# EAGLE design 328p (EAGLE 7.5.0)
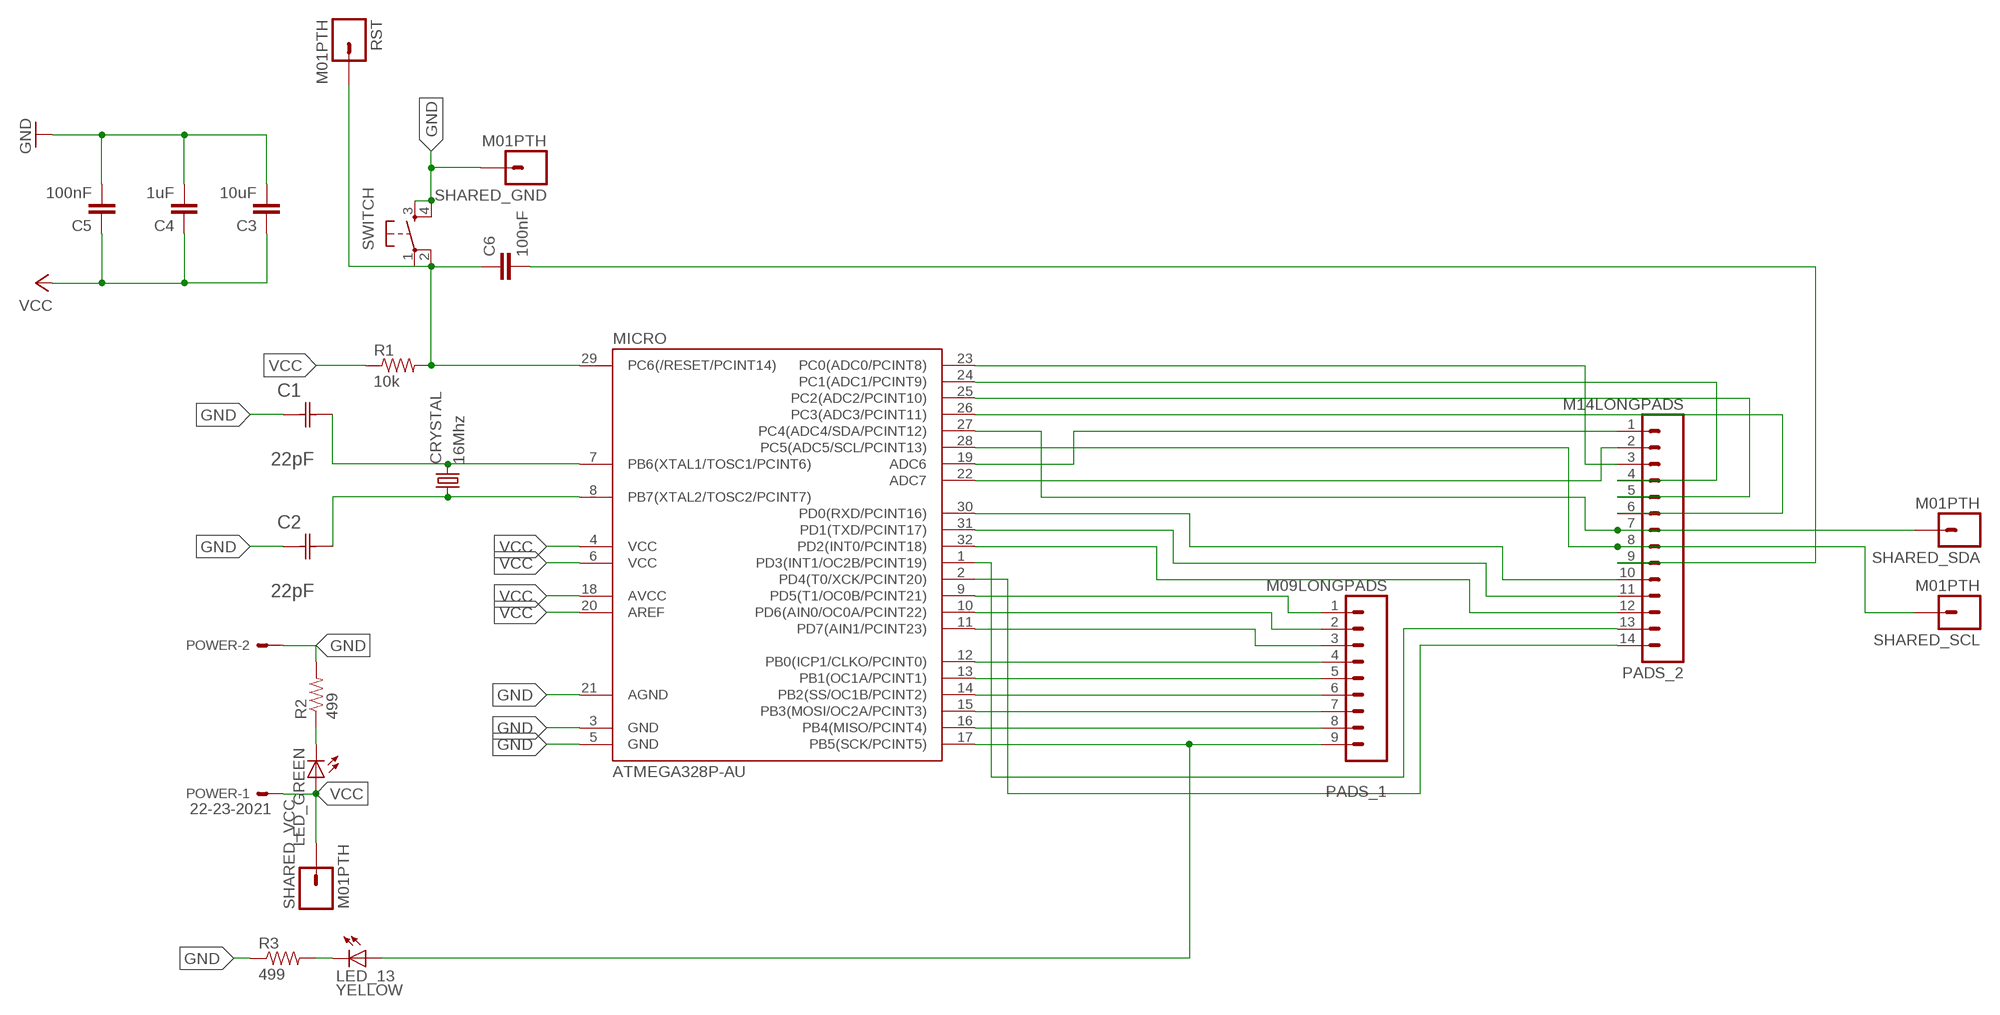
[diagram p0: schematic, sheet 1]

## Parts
C1  22pF  0612ZC225MAT2A  [CAPC3216X178N]
C2  22pF  0612ZC225MAT2A  [CAPC3216X178N]
C3  10uF  CAP1206  [1206]
C4  1uF  CAP1206  [1206]
C5  100nF  CAP1206  [1206]
C6  100nF  CAP1206  [1206]
CRYSTAL  16Mhz  CSM-7X-DU  [CSM-7X-DU]
LED_13  YELLOW  LED1206  [1206]
LED_GREEN  LED1206  [1206]
MICRO  ATMEGA328P-AU  ATMEGA48/88/168-AU  [TQFP32-08]
PADS_1  M09LONGPADS  [1X09_LONGPADS]
PADS_2  M14LONGPADS  [1X14-LONGPADS]
POWER  22-23-2021  [22-23-2021]
R1  10k  RESISTOR1206  [1206]
R2  499  RESISTOR1206  [1206]
R3  499  RESISTOR1206  [1206]
RST  M01PTH  [1X01]
SHARED_GND  M01PTH  [1X01]
SHARED_SCL  M01PTH  [1X01]
SHARED_SDA  M01PTH  [1X01]
SHARED_VCC  M01PTH  [1X01]
SWITCH  6MM_SWITCH6MM_SWITCH  [6MM_SWITCH]

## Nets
GND: C1.1(C1) C2.1(C1) C3.2 C4.2 C5.2 MICRO.3(GND) MICRO.5(GND) MICRO.21(AGND) POWER.2 R2.2 R3.1 SHARED_GND.1 SWITCH.3(S) SWITCH.4(S1)
N$1: MICRO.9(PD5(T1/OC0B/PCINT21)) PADS_1.1
N$2: C1.2(C2) CRYSTAL.2 MICRO.7(PB6(XTAL1/TOSC1/PCINT6))
N$3: C6.2 PADS_2.9
N$4: MICRO.10(PD6(AIN0/OC0A/PCINT22)) PADS_1.2
N$5: MICRO.11(PD7(AIN1/PCINT23)) PADS_1.3
N$6: MICRO.12(PB0(ICP1/CLKO/PCINT0)) PADS_1.4
N$7: MICRO.13(PB1(OC1A/PCINT1)) PADS_1.5
N$8: MICRO.14(PB2(SS/OC1B/PCINT2)) PADS_1.6
N$9: C2.2(C2) CRYSTAL.1 MICRO.8(PB7(XTAL2/TOSC2/PCINT7))
N$10: MICRO.15(PB3(MOSI/OC2A/PCINT3)) PADS_1.7
N$11: MICRO.16(PB4(MISO/PCINT4)) PADS_1.8
N$12: LED_13.1(A) MICRO.17(PB5(SCK/PCINT5)) PADS_1.9
N$13: MICRO.19(ADC6) PADS_2.1
N$14: MICRO.22(ADC7) PADS_2.2
N$15: MICRO.23(PC0(ADC0/PCINT8)) PADS_2.3
N$16: MICRO.24(PC1(ADC1/PCINT9)) PADS_2.4
N$17: MICRO.25(PC2(ADC2/PCINT10)) PADS_2.5
N$18: MICRO.26(PC3(ADC3/PCINT11)) PADS_2.6
N$19: MICRO.27(PC4(ADC4/SDA/PCINT12)) PADS_2.7 SHARED_SDA.1
N$20: MICRO.30(PD0(RXD/PCINT16)) PADS_2.10
N$21: MICRO.31(PD1(TXD/PCINT17)) PADS_2.11
N$22: MICRO.32(PD2(INT0/PCINT18)) PADS_2.12
N$23: MICRO.1(PD3(INT1/OC2B/PCINT19)) PADS_2.13
N$24: MICRO.2(PD4(T0/XCK/PCINT20)) PADS_2.14
N$25: MICRO.28(PC5(ADC5/SCL/PCINT13)) PADS_2.8 SHARED_SCL.1
N$26: LED_GREEN.2(C) R2.1
N$27: LED_13.2(C) R3.2
N$28: C6.1 MICRO.29(PC6(/RESET/PCINT14)) R1.2 RST.1 SWITCH.1(P) SWITCH.2(P1)
VCC: C3.1 C4.1 C5.1 LED_GREEN.1(A) MICRO.4(VCC) MICRO.6(VCC) MICRO.18(AVCC) MICRO.20(AREF) POWER.1 R1.1 SHARED_VCC.1

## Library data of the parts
C1 C2 = AVX_By_element14_Batch_1:0612ZC225MAT2A: Capacitor 1206; MPN: 0612ZC225MAT2A; OC_FARNELL: -; OC_NEWARK: 12N3209; SUPPLIER: AVX; TOLERANCE: ±20%; VALUE: 2.2µF; VOLTAGERATING: 10V
C3-C6 = 01_SparkFun:CAP: Capacitor
CRYSTAL = 01_FAB_Hello:CSM-7X-DU: SMD CRYSTAL; OC_FARNELL: unknown; OC_NEWARK: unknown
LED_13 LED_GREEN = 01_FAB_Hello:LED
MICRO = atmega8:ATMEGA48/88/168
PADS_1 = 01_SparkFun:M09: Header 9 Standard 9-pin 0.1" header. Use with straight break away headers (SKU : PRT-00116), right angle break away headers (PRT-00553), swiss pins (PRT-00743), machine pins (PRT-00117), and female headers (PRT-00115).
PADS_2 = 01_SparkFun:M14: Header 14 Standard 14-pin 0.1" header. Use with straight break away headers (SKU : PRT-00116), right angle break away headers (PRT-00553), swiss pins (PRT-00743), machine pins (PRT-00117), and female headers (PRT-00115).
POWER = con-molex:22-23-2021: .100" (2.54mm) Center Header - 2 Pin; MF: MOLEX; MPN: 22-23-2021; OC_FARNELL: 1462926; OC_NEWARK: 25C3832
R1-R3 = 01_SparkFun:RESISTOR: Resistor
RST SHARED_GND SHARED_SCL SHARED_SDA SHARED_VCC = 01_SparkFun:M01: Header 1
SWITCH = 01_FAB_Hello:6MM_SWITCH: OMRON SWITCH

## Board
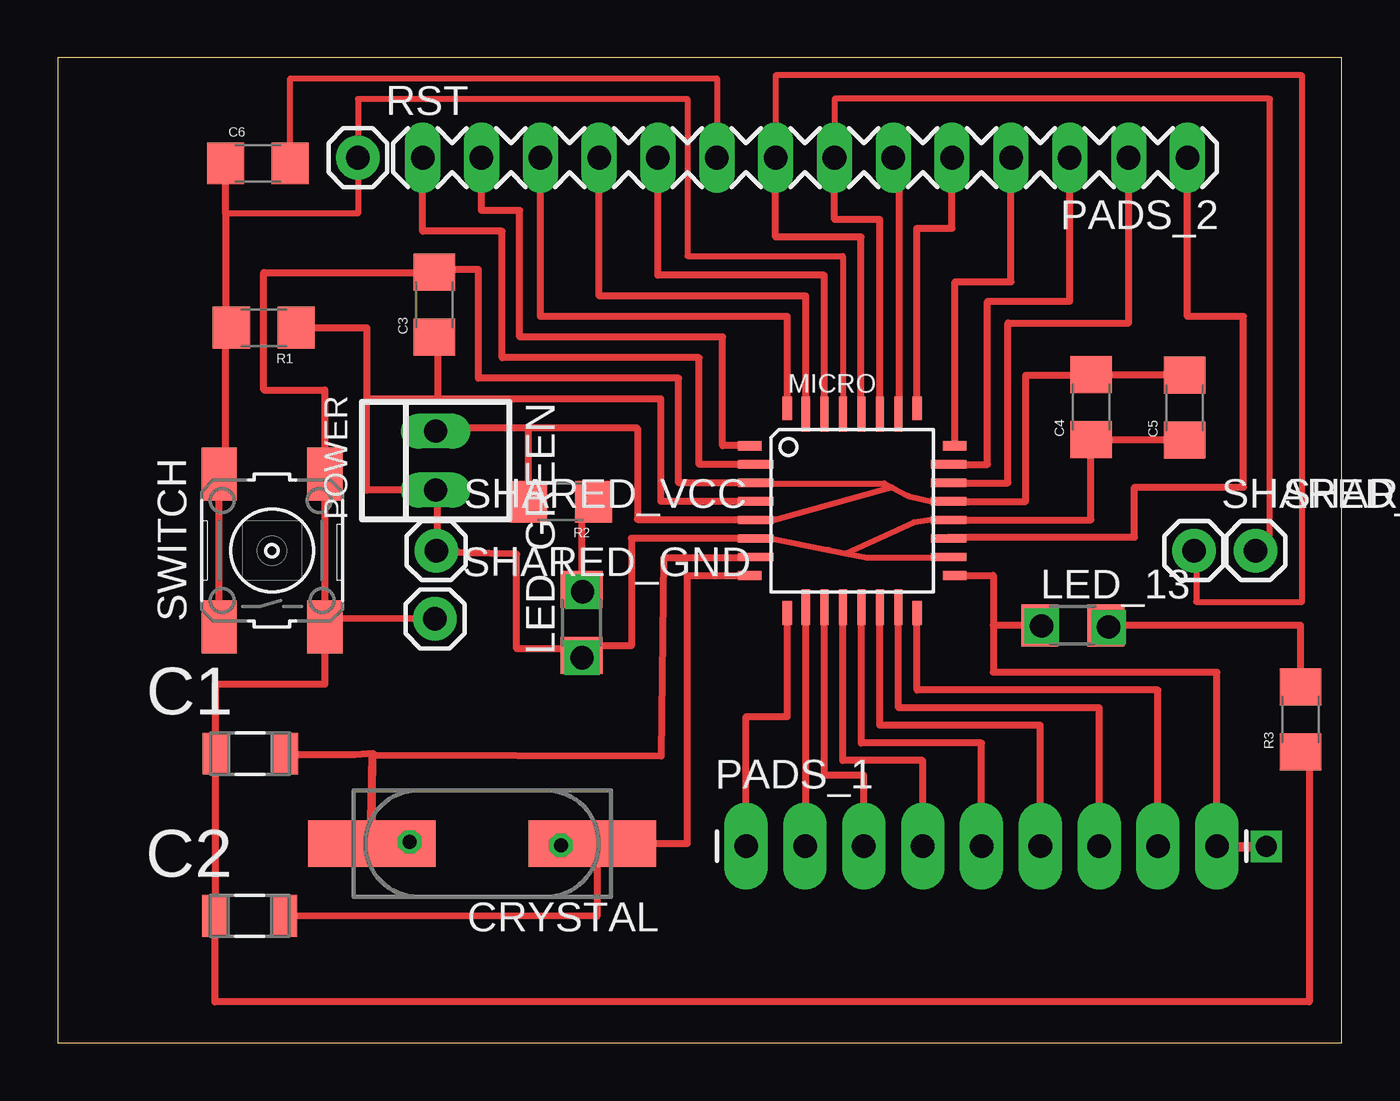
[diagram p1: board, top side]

Size 55.42 x 42.54 mm. Coordinates in mm from the lower left corner, seen from the top.
Outline: 0,0 55.42,0 55.42,42.54 0,42.54 0,0
Copper layers (1*16): Top 0.035mm / dielectric 1.5mm / Bottom 0.035mm
Design rules "default": minimum track width 10mil, minimum drill 24mil, track to track 8mil, track to pad 8mil, pad to pad 8mil, via to via 8mil, smd to smd 8mil, copper to edge 40mil, drill to drill 8mil, minimum pad ring 10mil, minimum via ring 8mil, stop-mask expansion 4mil, vias tented up to drill 0mil, thermal gap 10mil

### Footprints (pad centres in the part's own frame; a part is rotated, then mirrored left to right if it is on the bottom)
CAPC3216X178N = smd 1.118 x 1.803: 1 -1.499,0; 2 1.499,0
1206 = smd 1.6 x 1.8: 1 -1.4,0; 2 1.4,0
CSM-7X-DU = smd 5.5 x 2: 1 -4.75,0; 2 4.75,0
1206' = smd 1.6 x 1.803: 1 -1.422,0; 2 1.422,0
TQFP32-08 = smd 1.016 x 0.406: 1 -4.42,2.8; 8 -4.42,-2.8; 17 4.42,-2.8; 24 4.42,2.8 | smd 1.524 x 0.356: 2 -4.166,2; 3 -4.166,1.2; 4 -4.166,0.4; 5 -4.166,-0.4; 6 -4.166,-1.2; 7 -4.166,-2; 18 4.166,-2; 19 4.166,-1.2; 20 4.166,-0.4; 21 4.166,0.4; 22 4.166,1.2; 23 4.166,2 | smd 0.406 x 1.016: 9 -2.8,-4.42; 16 2.8,-4.42; 25 2.8,4.42; 32 -2.8,4.42 | smd 0.356 x 1.524: 10 -2,-4.166; 11 -1.2,-4.166; 12 -0.4,-4.166; 13 0.4,-4.166; 14 1.2,-4.166; 15 2,-4.166; 26 2,4.166; 27 1.2,4.166; 28 0.4,4.166; 29 -0.4,4.166; 30 -1.2,4.166; 31 -2,4.166
1X09_LONGPADS = drill 1.016 pad 1.88 long: 1 0,0; 2 2.54,0; 3 5.08,0; 4 7.62,0; 5 10.16,0; 6 12.7,0; 7 15.24,0; 8 17.78,0; 9 20.32,0
1X14-LONGPADS = drill 1.016 long: 1 0,0; 2 2.54,0; 3 5.08,0; 4 7.62,0; 5 10.16,0; 6 12.7,0; 7 15.24,0; 8 17.78,0; 9 20.32,0; 10 22.86,0; 11 25.4,0; 12 27.94,0; 13 30.48,0; 14 33.02,0
22-23-2021 = drill 1 long: 1 -1.27,0; 2 1.27,0
1X01 = drill 1.016 pad 1.88: 1 0,0
6MM_SWITCH = smd 2.286 x 1.524: 1 -3.302,2.286; 2 3.302,2.286; 3 -3.302,-2.286; 4 3.302,-2.286

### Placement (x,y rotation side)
C1  8.31,12.5 0 top
C2  8.28,5.49 0 top
C3  16.26,31.88 90 top
C4  44.6,27.46 90 top
C5  48.64,27.43 90 top
C6  8.64,37.97 0 top
CRYSTAL  18.31,8.61 180 top
LED_13  YELLOW  [1206']  43.81,18.03 0 top
LED_GREEN  [1206']  22.61,18.16 90 top
MICRO  34.29,22.99 0 top
PADS_1  29.72,8.51 0 top
PADS_2  48.77,38.23 180 top
POWER  16.31,25.15 90 top
R1  8.89,30.89 180 top
R2  21.72,23.37 180 top
R3  53.64,13.97 90 top
RST  12.95,38.23 0 top
SHARED_GND  16.28,18.31 0 top
SHARED_SCL  49.05,21.26 0 top
SHARED_SDA  51.71,21.26 0 top
SHARED_VCC  16.33,21.26 0 top
SWITCH  9.25,21.26 90 top

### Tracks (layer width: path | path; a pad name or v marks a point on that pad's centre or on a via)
GND
  Top 0.254: MICRO.3 30.15,24.16 35.68,24.16 | 35.68,24.16 36.7,23.62 37.85,23.37 | 30.73,22.61 30.99,22.61 35.86,23.95 | 35.86,23.95 36,23.99 | 35.68,24.16 35.86,23.95
  Top 0.305: MICRO.5 | MICRO.21 | 6.68,5.49 C2.1 6.78,1.78 54.03,1.78 54.03,12.57 R3.1 | 20.83,23.88 R2.2 20.83,24.13 | 20.83,23.88 | MICRO.5 30.12,22.61 25.02,22.61 25.02,26.54 20.32,26.54 | 30.73,22.61 MICRO.5 | MICRO.21 37.85,23.37 | MICRO.3 26.8,24.19 26.8,28.7 18.16,28.7 18.16,33.4 16.26,33.4 C3.2 8.89,33.27 8.89,28.19 11.53,28.19 SWITCH.4 11.53,18.34 | 6.73,5.97 6.81,5.97 C1.1 | C1.1 6.73,12.5 | 20.32,23.88 20.19,23.88 | 20.32,26.54 16.31,26.54 POWER.2 | 20.83,23.88 20.32,23.88 | 20.32,23.88 20.32,26.54 | 6.86,12.5 C1.1 | C1.1 6.81,15.49 11.53,15.49 SWITCH.3 11.53,18.34 | SHARED_GND.1 11.53,18.34 | MICRO.21 41.78,23.39 41.78,28.83 44.6,28.83 C4.2 48.64,28.86 C5.2
  Top 0.406: C2.1 6.73,5.49 | 6.73,5.49 6.73,5.46 | 6.73,5.49 6.73,5.97
N$1
  Top 0.305: PADS_1.1 29.72,14.1 31.49,14.1 MICRO.9
N$2
  Top 0.305: MICRO.7 30.12,20.95 26.16,20.95 26.06,12.4 13.56,12.45 13.49,8.61 CRYSTAL.2 13.61,12.5 12.83,12.45 9.8,12.45 C1.2
N$3
  Top 0.254: C6.2 10.03,41.66 28.45,41.66 PADS_2.9
N$4
  Top 0.305: PADS_1.2 32.29,8.51 MICRO.10
N$5
  Top 0.305: PADS_1.3 34.8,11.56 33.09,11.56 MICRO.11
N$6
  Top 0.305: 33.91,18.82 MICRO.12 33.89,12.19 37.34,12.19 PADS_1.4
N$7
  Top 0.305: MICRO.13 34.69,12.95 39.88,12.95 PADS_1.5
N$8
  Top 0.305: MICRO.14 35.49,13.72 42.42,13.72 PADS_1.6
N$9
  Top 0.305: 9.78,5.46 C2.2 | MICRO.8 27.18,20.19 27.18,8.61 CRYSTAL.1 23.27,8.61 23.27,5.46 C2.2 | C2.2
N$10
  Top 0.305: PADS_1.7 44.96,14.48 36.29,14.48 MICRO.15
N$11
  Top 0.305: MICRO.16 37.09,15.24 47.5,15.24 PADS_1.8
N$12
  Top 0.305: 40.39,18.03 40.39,16 50.04,16 PADS_1.9 | LED_13.1 40.39,18.03 | MICRO.17 40.39,20.19 40.39,18.03
N$13
  Top 0.305: MICRO.19 38.46,21.84 46.48,21.84 46.48,24 51.18,24 51.18,31.37 48.77,31.37 PADS_2.1
N$14
  Top 0.305: MICRO.22 41.02,24.19 41.02,31.09 46.23,31.09 PADS_2.2
N$15
  Top 0.305: MICRO.23 40.13,24.99 40.13,32.03 43.69,32.03 PADS_2.3
N$16
  Top 0.305: PADS_2.4 41.15,32.87 38.73,32.87 38.73,25.79 MICRO.24
N$17
  Top 0.305: MICRO.25 37.08,35.18 38.61,35.18 PADS_2.5
N$18
  Top 0.305: MICRO.26 36.32,27.15 36.32,37.34 arc-90 36.07,37.59 PADS_2.6
N$19
  Top 0.254: PADS_2.7 33.53,40.77 52.32,40.77 52.32,21.29 51.71,21.29 SHARED_SDA.1
  Top 0.305: MICRO.27 35.49,35.56 33.53,35.56 PADS_2.7
N$20
  Top 0.305: MICRO.30 33.09,33.15 25.91,33.15 PADS_2.10
N$21
  Top 0.305: MICRO.31 32.29,32.26 23.37,32.26 PADS_2.11
N$22
  Top 0.305: PADS_2.12 20.83,31.37 31.5,31.37 MICRO.32
N$23
  Top 0.305: MICRO.1 28.7,25.79 28.7,30.48 19.94,30.48 19.94,35.94 18.29,35.94 PADS_2.13
N$24
  Top 0.305: MICRO.2 27.69,24.99 27.69,29.59 19.18,29.59 19.18,35.05 15.75,35.05 PADS_2.14
N$25
  Top 0.254: SHARED_SCL.1 49.15,21.26 49.15,19.05 53.72,19.05 53.72,41.78 30.99,41.78 PADS_2.8
  Top 0.305: MICRO.28 34.67,27.15 34.67,34.8 30.99,34.8 PADS_2.8
N$26
  Top 0.305: 23.49,23.75 R2.1 22.61,23.62 LED_GREEN.2
N$27
  Top 0.305: LED_13.2 53.65,18.03 R3.2
N$28
  Top 0.254: MICRO.29 33.89,33.98 27.18,33.98 27.18,40.77 12.95,40.77 RST.1 12.95,35.81 7.24,35.81
  Top 0.305: C6.1 7.24,35.81 7.24,31.5 | 7.24,31.5 7.49,31.5 R1.2 | SWITCH.1 SWITCH.2 7.49,24.64 7.24,24.64 7.24,31.5
N$29  (via drill 0.6)
  other vias: 15.19,8.69
N$30  (via drill 0.6)
  other vias: 21.72,8.53
N$31  (via drill 1)
  other vias: 22.66,19.48
N$32  (via drill 1)
  other vias: 22.63,16.64
N$33  (via drill 1)
  other vias: 42.47,18.01
N$34  (via drill 1)
  other vias: 45.36,17.96
N$35  (via drill 0.9)
  other vias: 52.17,8.48
N$36
  Top 0.406: 50.06,8.46 52.27,8.46 52.27,8.36
VCC
  Top 0.254: 30.81,21.79 33.27,21.29 34.02,21.14 | 34.02,21.14 34.92,20.95 38.46,20.95 | MICRO.20 37.85,22.59 37.85,22.61 36.96,22.48 34.02,21.14
  Top 0.305: MICRO.18 38.46,20.95 | MICRO.20 | MICRO.4 26.03,23.39 26.03,27.81 16.38,27.81 | 16.38,27.81 13.34,27.81 | LED_GREEN.1 22.61,17.14 22.73,17.14 | MICRO.20 37.85,22.61 | 30.81,21.79 MICRO.6 24.77,21.79 24.77,17.14 22.73,17.14 | R1.1 13.34,30.89 13.34,27.81 | C3.1 16.38,30.48 16.38,27.81 | 13.34,27.81 13.34,23.88 POWER.1 16.38,23.85 | 16.38,23.85 17.27,23.88 | 17.27,21.21 SHARED_VCC.1 17.12,21.26 16.38,21.18 | 22.73,17.14 22.73,17.02 19.81,17.02 19.81,21.11 16.38,21.18 | 16.38,21.18 16.38,23.85 | MICRO.20 44.6,22.59 C4.1 48.64,26.06 C5.1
